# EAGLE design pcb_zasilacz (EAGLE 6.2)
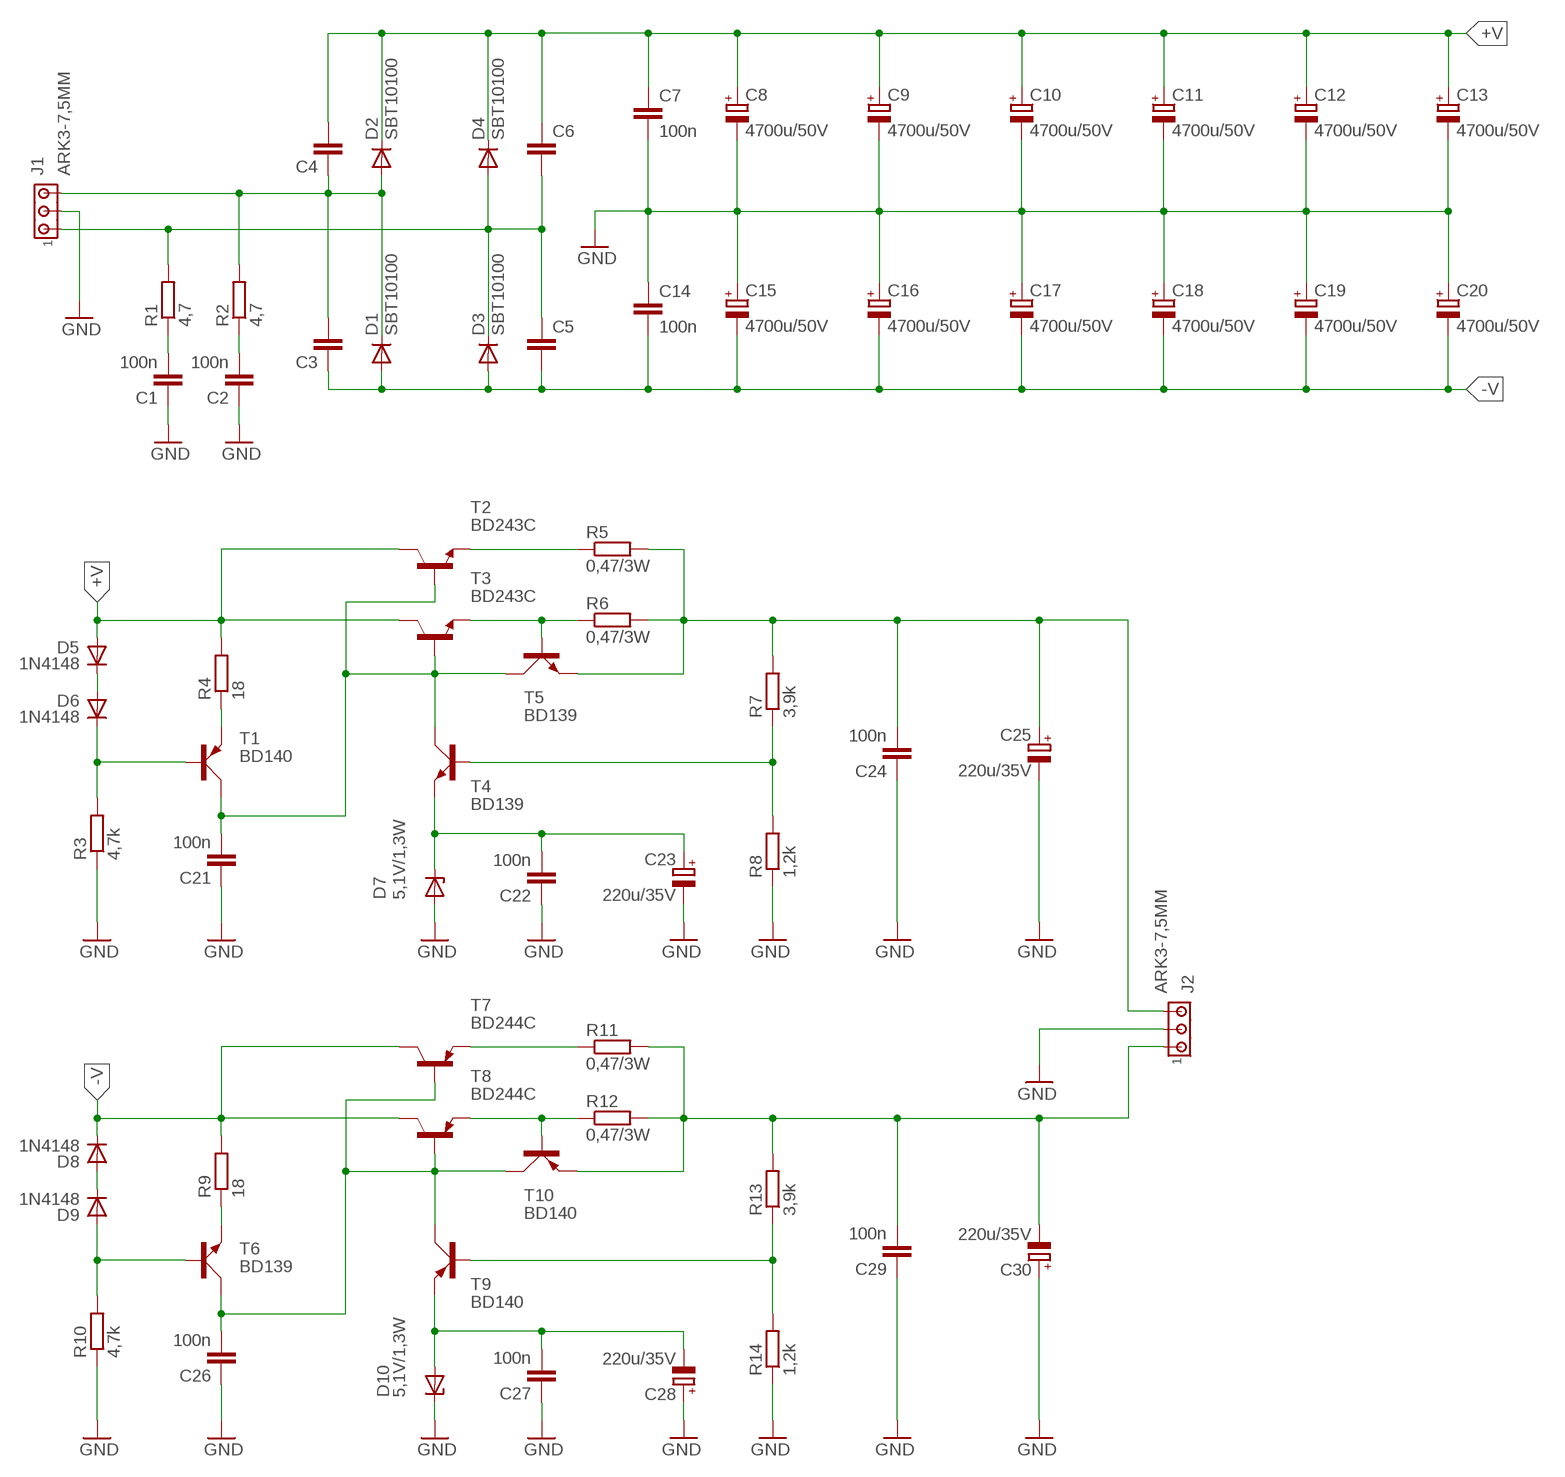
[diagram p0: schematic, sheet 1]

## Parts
C1  100n  C-EU050-025X075  [C050-025X075]
C2  100n  C-EU050-025X075  [C050-025X075]
C3  C-EU050-025X075  [C050-025X075]
C4  C-EU050-025X075  [C050-025X075]
C5  C-EU050-025X075  [C050-025X075]
C6  C-EU050-025X075  [C050-025X075]
C7  100n  C-EU050-025X075  [C050-025X075]
C8  4700u/50V  CPOL-EUE10-22.5  [EB22,5D]
C9  4700u/50V  CPOL-EUE10-22.5  [EB22,5D]
C10  4700u/50V  CPOL-EUE10-22.5  [EB22,5D]
C11  4700u/50V  CPOL-EUE10-22.5  [EB22,5D]
C12  4700u/50V  CPOL-EUE10-22.5  [EB22,5D]
C13  4700u/50V  CPOL-EUE10-22.5  [EB22,5D]
C14  100n  C-EU050-025X075  [C050-025X075]
C15  4700u/50V  CPOL-EUE10-22.5  [EB22,5D]
C16  4700u/50V  CPOL-EUE10-22.5  [EB22,5D]
C17  4700u/50V  CPOL-EUE10-22.5  [EB22,5D]
C18  4700u/50V  CPOL-EUE10-22.5  [EB22,5D]
C19  4700u/50V  CPOL-EUE10-22.5  [EB22,5D]
C20  4700u/50V  CPOL-EUE10-22.5  [EB22,5D]
C21  100n  C-EU050-025X075  [C050-025X075]
C22  100n  C-EU050-025X075  [C050-025X075]
C23  220u/35V  CPOL-EUE3.5-8  [E3,5-8]
C24  100n  C-EU050-025X075  [C050-025X075]
C25  220u/35V  CPOL-EUE3.5-8  [E3,5-8]
C26  100n  C-EU050-025X075  [C050-025X075]
C27  100n  C-EU050-025X075  [C050-025X075]
C28  220u/35V  CPOL-EUE3.5-8  [E3,5-8]
C29  100n  C-EU050-025X075  [C050-025X075]
C30  220u/35V  CPOL-EUE3.5-8  [E3,5-8]
D1  SBT10100  DIODE-TO220V  [TO220ACS]
D2  SBT10100  DIODE-TO220V  [TO220ACS]
D3  SBT10100  DIODE-TO220V  [TO220ACS]
D4  SBT10100  DIODE-TO220V  [TO220ACS]
D5  1N4148  DIODE-DO34-7  [DO34-7]
D6  1N4148  DIODE-DO34-7  [DO34-7]
D7  5,1V/1,3W  ZENER-DIODEDO41Z10  [DO41Z10]
D8  1N4148  DIODE-DO34-7  [DO34-7]
D9  1N4148  DIODE-DO34-7  [DO34-7]
D10  5,1V/1,3W  ZENER-DIODEDO41Z10  [DO41Z10]
J1  ARK3-7,5MM  [3PIN-7,5MM]
J2  ARK3-7,5MM  [3PIN-7,5MM]
R1  4,7  R-EU_0207/7  [0207/7]
R2  4,7  R-EU_0207/7  [0207/7]
R3  4,7k  R-EU_0207/7  [0207/7]
R4  18  R-EU_0207/7  [0207/7]
R5  0,47/3W  R-EU_0617/17  [0617/17]
R6  0,47/3W  R-EU_0617/17  [0617/17]
R7  3,9k  R-EU_0207/7  [0207/7]
R8  1,2k  R-EU_0207/7  [0207/7]
R9  18  R-EU_0207/7  [0207/7]
R10  4,7k  R-EU_0207/7  [0207/7]
R11  0,47/3W  R-EU_0617/17  [0617/17]
R12  0,47/3W  R-EU_0617/17  [0617/17]
R13  3,9k  R-EU_0207/7  [0207/7]
R14  1,2k  R-EU_0207/7  [0207/7]
T1  BD140  [TO126AV]
T2  BD243C  -NPN-TO220V  [TO220V]
T3  BD243C  -NPN-TO220V  [TO220V]
T4  BD139  [TO126AV]
T5  BD139  [TO126AV]
T6  BD139  [TO126AV]
T7  BD244C  -PNP-TO220V  [TO220V]
T8  BD244C  -PNP-TO220V  [TO220V]
T9  BD140  [TO126AV]
T10  BD140  [TO126AV]

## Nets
+V: C4.2 C6.1 C7.1 C8.+ C9.+ C10.+ C11.+ C12.+ C13.+ D2.C D4.C D5.A R4.2 T2.2(C) T3.2(C)
-V: C3.1 C5.2 C14.2 C15.- C16.- C17.- C18.- C19.- C20.- D1.A D3.A D8.C R9.2 T7.2(C) T8.2(C)
GND: C1.1 C2.1 C7.2 C8.- C9.- C10.- C11.- C12.- C13.- C14.1 C15.+ C16.+ C17.+ C18.+ C19.+ C20.+ C21.1 C22.1 C23.- C24.1 C25.- C26.1 C27.1 C28.+ C29.1 C30.+ D7.A D10.C J1.P2 J2.P2 R3.1 R8.1 R10.1 R14.1
N$1: C22.2 C23.+ D7.C T4.E
N$2: R5.1 T2.3(E)
N$3: C1.2 R1.1
N$4: D5.C D6.A
N$5: R7.1 R8.2 T4.B
N$6: C27.2 C28.- D10.A T9.E
N$7: D6.C R3.2 T1.B
N$8: C2.2 R2.1
N$9: C3.2 C4.1 D1.C D2.A J1.P3 R2.2
N$10: C5.1 C6.2 D3.C D4.A J1.P1 R1.2
N$11: R4.1 T1.E
N$12: C21.2 T1.C T2.1(B) T3.1(B) T4.C T5.C
N$13: R6.1 T3.3(E) T5.B
N$14: R13.1 R14.2 T9.B
N$15: C24.2 C25.+ J2.P3 R5.2 R6.2 R7.2 T5.E
N$16: D8.A D9.C
N$17: D9.A R10.2 T6.B
N$18: R9.1 T6.E
N$19: C26.2 T6.C T7.1(B) T8.1(B) T9.C T10.C
N$20: R11.1 T7.3(E)
N$21: R12.1 T8.3(E) T10.B
N$22: C29.2 C30.- J2.P1 R11.2 R12.2 R13.2 T10.E

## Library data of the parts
C1-C7 C14 C21 C22 C24 C26 C27 C29 = rcl:C-EU: CAPACITOR, European symbol
C8-C13 C15-C20 C23 C25 C28 C30 = rcl:CPOL-EU: POLARIZED CAPACITOR, European symbol
D1-D6 D8 D9 = diode:DIODE-: DIODE
D7 D10 = diode:ZENER-DIODE: Z-Diode
J1 J2 = zlacza_futrzak:ARK3: ARK 3 Raster 5mm i 3,5mm
R1-R14 = rcl:R-EU_: RESISTOR, European symbol
T1 T9 T10 = transistor-power:BD140: PNP TRANSISTOR
T2 T3 = transistor:*-NPN-: NPN Transistror BF959 corrected 2008.03.06
T4-T6 = transistor-power:BD139: NPN TRANSISTOR
T7 T8 = transistor:*-PNP-: PNP Transistror

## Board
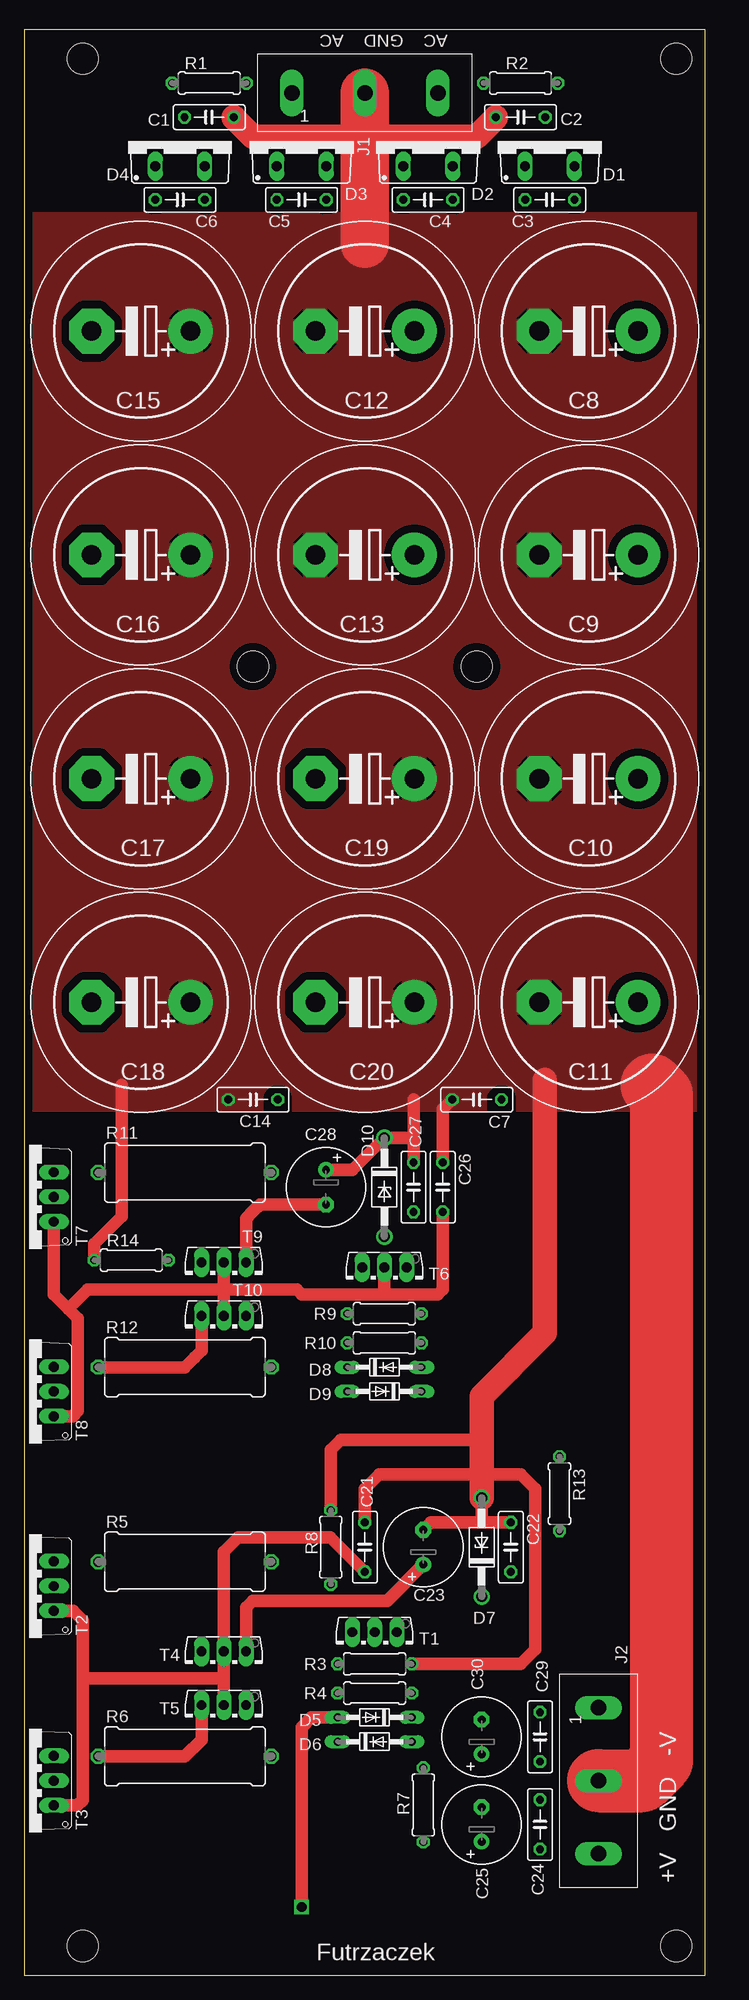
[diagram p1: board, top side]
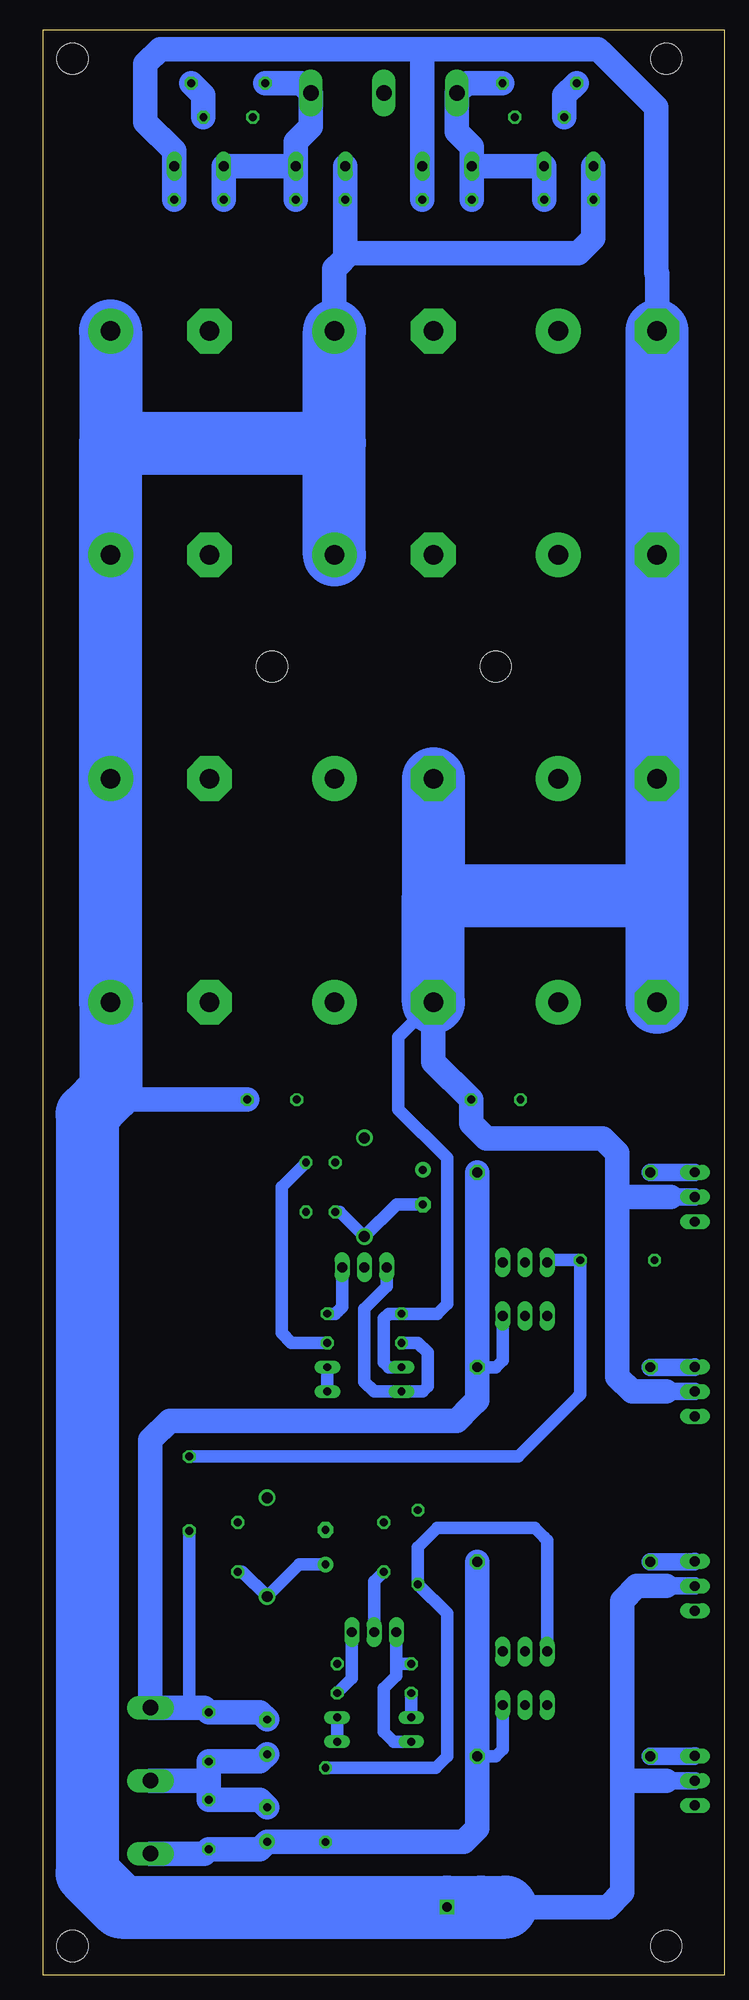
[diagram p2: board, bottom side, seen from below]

Size 70 x 200 mm. Coordinates in mm from the lower left corner, seen from the top.
Outline: 0,0 70,0 70,200 0,200 0,0
Copper layers (1*16): Top 0.035mm / dielectric 1.5mm / Bottom 0.035mm
Design rules: minimum track width 10mil, minimum drill 23mil, track to track 8mil, track to pad 8mil, pad to pad 8mil, via to via 8mil, smd to smd 8mil, copper to edge 20mil, drill to drill 8mil, minimum pad ring 10mil, minimum via ring 8mil, stop-mask expansion 4mil, vias tented up to drill 0mil, thermal gap 10mil
Holes 3.2 mm at 67,197 6,197 6,3 67,3 46.5,134.5 23.5,134.5

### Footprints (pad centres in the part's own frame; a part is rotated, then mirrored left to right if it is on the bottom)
C050-025X075 = drill 0.813 octagon: 1 -2.54,0; 2 2.54,0
EB22,5D = drill 2.007 pad 4.597: + -5.08,0 | drill 2.007 pad 4.597 octagon: - 5.08,0
E3,5-8 = drill 0.813 pad 1.6: + -1.778,0 | drill 0.813 pad 1.6 octagon: - 1.778,0
TO220ACS = drill 1.016 long: A 2.54,-2.54; C -2.54,-2.54
DO34-7 = drill 0.813 long: A 3.81,0; C -3.81,0
DO41Z10 = drill 1.118: A 5.08,0; C -5.08,0
3PIN-7,5MM = drill 1.6 long: P1 -7.5,0; P2 0,0; P3 7.5,0
0207/7 = drill 0.813 octagon: 1 -3.81,0; 2 3.81,0
0617/17 = drill 1.016 octagon: 1 -8.89,0; 2 8.89,0
TO126AV = drill 1.016 long: B 2.286,-1.27; C 0,-1.27; E -2.286,-1.27
TO220V = drill 1.016 long: 1 -2.54,-2.54; 2 0,-2.54; 3 2.54,-2.54

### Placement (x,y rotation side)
C1  19,191 180 top
C2  51,191 0 top
C3  54,182.5 180 top
C4  41.5,182.5 180 top
C5  28.5,182.5 0 top
C6  16,182.5 0 top
C7  46.5,90 180 top
C8  58,169 180 top
C9  58,146 180 top
C10  58,123 180 top
C11  58,100 180 top
C12  35,169 180 top
C13  35,146 180 top
C14  23.5,90 0 top
C15  12,169 180 top
C16  12,146 180 top
C17  12,123 180 top
C18  12,100 180 top
C19  35,123 180 top
C20  35,100 180 top
C21  35,44 270 top
C22  50,44 270 top
C23  41,44 90 top
C24  53,15.5 270 top
C25  47,15.5 90 top
C26  43,81 270 top
C27  40,81 270 top
C28  31,81 270 top
C29  53,24.5 90 top
C30  47,24.5 90 top
D1  54,188.5 0 top
D2  41.5,188.5 0 top
D3  28.5,188.5 0 top
D4  16,188.5 0 top
D5  36,26.5 180 top
D6  36,24 0 top
D7  47,44 90 top
D8  37,62.5 0 top
D9  37,60 180 top
D10  37,81 270 top
J1  35,193.5 0 top
J2  59,20 270 top
R1  19,194.5 0 top
R2  51,194.5 180 top
R3  36,32 180 top
R4  36,29 180 top
R5  16.5,42.5 0 top
R6  16.5,22.5 0 top
R7  41,17.5 270 top
R8  31.5,44 270 top
R9  37,68 180 top
R10  37,65 180 top
R11  16.5,82.5 0 top
R12  16.5,62.5 0 top
R13  55,49.5 270 top
R14  11,73.5 0 top
T1  36,34 180 top
T2  0.5,40 90 top
T3  0.5,20 90 top
T4  20.5,32 180 top
T5  20.5,26.5 180 top
T6  37,71.5 180 top
T7  0.5,80 90 top
T8  0.5,60 90 top
T9  20.5,72 180 top
T10  20.5,66.5 180 top

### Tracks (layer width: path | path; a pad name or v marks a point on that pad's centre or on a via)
+V  (via drill 1)
  Top 1.27: D5.A 29.5,26.5 28.5,25.5 v28.5,7
  Bottom 1.27: D5.A R4.2
  Bottom 1.778: 6,40 T2.2 | T3.2 6,20
  Bottom 2.54: C7.1 58.5,90 62.5,90 63.25,90.75 | D2.C C4.2 38.96,177 | 38.96,177 38.96,176.54 39.5,176 40.08,175.42 C12.+ | 38.96,177 15,177 13.46,178.54 C6.1 D4.C | 22.5,7 12,7 10.5,8.5 10.5,20 | 10.5,20 10.5,38.5 9,40 6,40 | 6,20 10.5,20
  Bottom 6.452: C13.+ 40.08,157.5 | 40.08,157.5 C12.+ | 63.08,157.5 C9.+ C10.+ C11.+ 63.08,90.92 63.25,90.75 65.5,88.5 65.5,10.5 62,7 v28.5,7 25,7 22.5,7 | 63.08,157.5 40.08,157.5 | C8.+ 63.08,157.5
-V
  Bottom 1.27: D8.C 34.5,62.5 35,63 35,67.5 34.5,68 R9.2 29.5,68 28.5,69 28.5,84 33.5,89 33.5,96.42 C20.-
  Bottom 1.778: 6,60 T8.2 | T7.2 5.5,80
  Bottom 2.54: C20.- 29.92,93.88 C14.2 26.04,87.54 24.5,86 12.5,86 11,84.5 11,80.5 | C5.2 D3.A 31.04,196.04 31.04,197.96 31,198 | C3.1 D1.A 56.54,187.54 59.5,190.5 59.5,196.5 58,198 33,198 31,198 | C15.- 6.92,174.92 7,175 7,192 12.5,197.5 | 12.5,197.5 13,198 | 31,198 13,198 | 13,198 12.5,197.5 | 11,80.5 11,61.5 9.5,60 6,60 | 5.5,80 10.5,80 11,80.5
  Bottom 6.452: C18.- 6.92,111 | 6.92,111 C17.- C16.- C15.- | C20.- 29.92,111 | 29.92,111 6.92,111 | C19.- 29.92,111
GND
  Top 1.27: R14.1 7.19,75.19 10,78 10,89.5 10,91.5 | C27.1 40,86 | 40,86 40,90 | 40,86 39.92,86.08 D10.C 33.7,82.78 C28.+ | C26.1 43,89.04 C7.2 | C22.1 47,46.54 | 47,46.54 D7.A | C23.- 41.76,46.54 47,46.54 | C21.1 35,50 36.5,51.5 47,51.5 51,51.5 52.5,50 52.5,33.5 51,32 R3.1 | R8.1 31.5,54 32.5,55 47,55
  Top 2.54: C2.1 48.46,190.96 47,189.5 46.5,189 35,189 23.5,189 21.54,190.96 C1.1 | D7.A 47,51.5 47,55 47,59.5 53.5,66 53.5,92
  Top 5: J1.P2 35,189 35,178
  Top 6.452: J2.P2 63.5,20 65.5,22 65.5,90.5 64.5,91.5
  Bottom 1.27: R10.1 44.5,65 45.5,66 45.5,80 45.5,81.04 C26.1
  Bottom 2.54: J2.P2 53,20 | 53,20 C29.1 47.76,21.96 C30.+ | C25.- 47.76,18.04 C24.1 53,20
  pour Top (isolate 0.813): 0,180 70,180 70,90 0,90
N$1
  Top 1.27: T4.E 22.79,36.79 22.79,37.79 23.5,38.5 37.28,38.5 C23.+
  Bottom 1.27: C22.2 49.54,41.46 D7.C 43.7,42.22 C23.+
N$2
  Bottom 1.778: R5.1 3.08,42.5 T2.3
N$3
  Bottom 2.54: C1.2 16.46,193.23 R1.1
N$4
  Bottom 1.27: D6.A D5.C
N$5
  Bottom 1.27: T4.B 18.21,44.71 18.5,45 19.5,46 29.5,46 31.5,44 R8.2 28.5,37.19 28.5,22.5 29.69,21.31 R7.1
N$6
  Top 1.27: T9.E 22.79,77.79 23.5,78.5 24.22,79.22 C28.-
  Bottom 1.27: C27.2 39.54,78.46 D10.A 33.7,79.22 C28.-
N$7
  Bottom 1.27: T1.B 33.71,32 | 33.71,32 33.71,30.79 35,29.5 35,25 34,24 D6.C | R3.2 33.71,32
N$8
  Bottom 2.54: C2.2 53.54,193.23 R2.1
N$9
  Bottom 2.54: C4.1 D2.A | C3.2 D1.C D2.A | D2.A 44.04,188.46 42.5,190 J1.P3 43.5,194.5 R2.2
N$10
  Bottom 2.54: C5.1 D3.C | C6.2 D4.A D3.C | D3.C 25.96,187.96 27.5,189.5 J1.P1 26.5,194.5 R1.2
N$11
  Bottom 1.27: T1.E 38.29,30.52 R4.1
N$12
  Top 1.27: T2.1 5.04,37.46 6,36.5 6,30.5 | 6,30.5 6,18 5.5,17.5 5.46,17.46 T3.1 | T5.C 20.5,30 20.5,30.5 | 20.5,30.5 6,30.5 | 20.5,30.5 T4.C 20.5,43.5 22,45 31.46,45 C21.2
  Bottom 1.27: T1.C 36,40.46 C21.2
N$13
  Top 1.27: T5.B 18.21,24.21 16.5,22.5 R6.1
  Bottom 1.778: R6.1 3.08,22.5 T3.3
N$14
  Bottom 1.27: T9.B 17.98,73.5 R14.2 14.81,59.69 15,59.5 21.19,53.31 R13.1
N$15
  Bottom 1.27: T5.E 22.79,23.21 23.5,22.5 R6.2 | R7.2 39.03,13.69 39,13.72
  Bottom 2.54: J2.P3 53.46,12.5 C24.2 47.76,12.96 C25.+ 39,13.72 26.78,13.72 25.5,15 25.39,15.11 R6.2 R5.2
N$16
  Bottom 1.27: D9.C D8.A
N$17
  Bottom 1.27: T6.B 34.71,70.79 37,68.5 37,66 37,65 37,61 36,60 D9.A 31,60 30.5,60.5 30.5,64 31.5,65 R10.2
N$18
  Bottom 1.27: R9.1 40,68 39.75,68.25 | 39.75,68.25 39.5,68.5 | T6.E 39.29,68.71 39.75,68.25
N$19
  Top 1.27: T7.1 3.04,69.96 4.5,68.5 | 4.5,68.5 5.5,67.5 5.5,58 4.96,57.46 T8.1 | T10.C 20.5,70.5 | 20.5,70.5 6.5,70.5 4.5,68.5 | 20.5,70.5 T9.C | T6.C 37,70.5 37,70 | 20.5,70.5 28,70.5 28.5,70 36.5,70 37,70 | 37,70 42.5,70 43,70.5 C26.2
N$20
  Bottom 1.778: R11.1 3.08,82.5 T7.3
N$21
  Top 1.27: R12.1 16.5,62.5 17.5,63.5 18.21,64.21 T10.B
  Bottom 1.778: R12.1 3.08,62.5 T8.3
N$22
  Bottom 1.27: R13.2 55,27.5 | 25.12,67.77 25.39,67.5 | T10.E 22.79,63.21 23.5,62.5 R12.2
  Bottom 2.54: R11.2 25.39,67.5 R12.2 25.39,59.11 26,58.5 27.5,57 57,57 59,55 J2.P1 55,27.5 53.46,27.5 C29.2 47.76,27.04 C30.-

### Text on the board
tPlace: AC GND AC | +V GND -V | Futrzaczek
